|   TEXAS INSTRUMENTS INCORPORATED
|   Standard Linear and Logic
|   IBIS Model of SN74LVTH16652
|   3.3-V ABT 16-BIT BUS TRANSCEIVERS AND REGISTERS
|   WITH 3-STATE OUTPUTS
|   TSSOP 56-pin package (DGG)
|   SSOP 56-pin package (DL)
[IBIS Ver]   3.2
[Comment char] |_char
[File Name]   sn74lvth16652.ibs
[File Rev]   1.1 | x_rev
[Date]   10/03/03
[Source]   File originated at Texas Instruments, Inc
[Notes]   The following is a sample IBIS file for the SN74LVTH16652.
|   - All test data contained in this file are derived from
|   actual measurement.
|   - The measurement used DGG package.
|   - We have data across voltage and temperature, but not across
|   process.
|   - Since this is a BiCMOS process, we have irregular trend for the
|   curves at high and low temperatures. This data was taken with
|   high temperature for strong case and low for weak case.
|   - Due to presence of BUS-HOLD at input, GND-CLAMP curves
|   have non-monotonic warnings.
|   - End point warning due to AC and DC mismatch.
|   - Due to the fact that the Device is 5-V Input/Output
|   tolarent, the I/O model has some Non-Monotonic Warnings.
|   - File created by Nobuhisa Ohtsubo, TIJ SLL Product Engineering.
|*   Property of Texas Instruments Incorporated.  Unauthorized   *
|*   reproduction and/or distribution is strictly prohibited.   *
|*   This product is protected under copyright law.   *
|*   Created 1998, (C) Copyright 1998, Texas Instruments Inc.,   *
|*   All Rights Reserved   *
|*   UNLESS THERE IS A SIGNED, WRITTEN AGREEMENT TO THE   *
|*   CONTRARY, TEXAS INSTRUMENTS ("TI") IS PROVIDING THE SPICE   *
|*   MODELS "AS IS" AND WITHOUT ANY WARRANTY, EXPRESSED OR   *
|*   IMPLIED.  TI assumes no liability for:   *
|*   1) the accuracy of the IBIS models provided to your   *
|*   company;   *
|*   2) the proper functioning of these IBIS models in your   *
|*   design or for any resulting applications; or   *
|*   3) infringement of patents, copyrights or intellectual   *
|*   property rights resulting from your use of these   *
|*   IBIS models.   *
|*   TI provides IBIS Models as a service to our customers.   *
|*   You and your company shall not distribute, sell or give   *
|*   these models to anyone else without prior written   *
|*   permission from TI.   *
|*   TI reserves the right to make changes to our products or   *
|*   to discontinue any semiconductor product or service   *
|*   without notice, and advises our customers to obtain the   *
|*   latest version of relevant information to verify, before   *
|*   placing orders, that the information being relied on is   *
|*   current.   *
|*   Please be aware that your receipt and use of the IBIS   *
|*   information provided shall serve as acceptance of these   *
|*   terms and conditions.  If you do not accept these terms,   *
|*   you should return or destroy the IBIS models and any   *
|*   other accompanying information immediately.   *
|   TSSOP PACKAGE (DGG)
[Component]   LVTH16652_DGG
[manufacturer]   Texas Instruments, Inc.
[Package]
|   typ   min   max
R_pkg   0.045   0.035   0.062
L_pkg   3.324nH   2.403nH   5.094nH
C_pkg   0.564pF   0.341pF   0.914nH
[Pin] signal_name   model_name   R_pin   L_pin   C_pin
1   1OEAB   LVTH16652_CTRL   0.062   5.094nH   0.856pF
2   1CLKAB   LVTH16652_CTRL   0.061   4.621nH   0.902pF
3   1SAB   LVTH16652_CTRL   0.060   4.316nH   0.802pF
4   GND   GND   0.059   3.968nH   0.698pF
5   1A1   LVTH16652_IO   0.057   3.716nH   0.649pF
6   1A2   LVTH16652_IO   0.042   3.517nH   0.652pF
7   VCC   POWER   0.041   3.160nH   0.570pF
8   1A3   LVTH16652_IO   0.039   2.981nH   0.482pF
9   1A4   LVTH16652_IO   0.039   2.809nH   0.447pF
10   1A5   LVTH16652_IO   0.038   2.715nH   0.409pF
11   GND   GND   0.041   2.675nH   0.391pF
12   1A6   LVTH16652_IO   0.039   2.536nH   0.366pF
13   1A7   LVTH16652_IO   0.039   2.457nH   0.348pF
14   1A8   LVTH16652_IO   0.038   2.411nH   0.353pF
15   2A1   LVTH16652_IO   0.039   2.456nH   0.355pF
16   2A2   LVTH16652_IO   0.039   2.471nH   0.349pF
17   2A3   LVTH16652_IO   0.040   2.580nH   0.370pF
18   GND   GND   0.038   2.651nH   0.389pF
19   2A4   LVTH16652_IO   0.038   2.739nH   0.411pF
20   2A5   LVTH16652_IO   0.039   2.838nH   0.449pF
21   2A6   LVTH16652_IO   0.038   2.988nH   0.484pF
22   VCC   POWER   0.038   3.105nH   0.564pF
23   2A7   LVTH16652_IO   0.040   3.427nH   0.638pF
24   2A8   LVTH16652_IO   0.056   3.654nH   0.641pF
25   GND   GND   0.057   3.932nH   0.700pF
26   2SAB   LVTH16652_CTRL   0.058   4.257nH   0.806pF
27   2CLKAB   LVTH16652_CTRL   0.057   4.580nH   0.914pF
28   2OEAB   LVTH16652_CTRL   0.059   5.038nH   0.861pF
29   2OEBA_BAR   LVTH16652_CTRL   0.060   5.058nH   0.858pF
30   2CLKBA   LVTH16652_CTRL   0.056   4.543nH   0.904pF
31   2SBA   LVTH16652_CTRL   0.057   4.240nH   0.803pF
32   GND   GND   0.057   3.929nH   0.700pF
33   2B8   LVTH16652_IO   0.056   3.616nH   0.637pF
34   2B7   LVTH16652_IO   0.037   3.368nH   0.640pF
35   VCC   POWER   0.036   3.024nH   0.563pF
36   2B6   LVTH16652_IO   0.035   2.876nH   0.474pF
37   2B5   LVTH16652_IO   0.035   2.745nH   0.444pF
38   2B4   LVTH16652_IO   0.037   2.683nH   0.405pF
39   GND   GND   0.038   2.603nH   0.382pF
40   2B3   LVTH16652_IO   0.038   2.510nH   0.362pF
41   2B2   LVTH16652_IO   0.036   2.412nH   0.341pF
42   2B1   LVTH16652_IO   0.038   2.416nH   0.349pF
43   1B8   LVTH16652_IO   0.037   2.403nH   0.349pF
44   1B7   LVTH16652_IO   0.037   2.429nH   0.341pF
45   1B6   LVTH16652_IO   0.036   2.482nH   0.358pF
46   GND   GND   0.037   2.615nH   0.381pF
47   1B5   LVTH16652_IO   0.035   2.669nH   0.402pF
48   1B4   LVTH16652_IO   0.036   2.763nH   0.442pF
49   1B3   LVTH16652_IO   0.036   2.942nH   0.478pF
50   VCC   POWER   0.035   3.053nH   0.564pF
51   1B2   LVTH16652_IO   0.036   3.409nH   0.641pF
52   1B1   LVTH16652_IO   0.058   3.698nH   0.641pF
53   GND   GND   0.059   3.975nH   0.697pF
54   1SBA   LVTH16652_CTRL   0.061   4.327nH   0.802pF
55   1CLKBA   LVTH16652_CTRL   0.061   4.624nH   0.905pF
56   1OEBA_BAR   LVTH16652_CTRL   0.060   5.063nH   0.858pF
|   SSOP PACKAGE (DL)
[Component]   LVTH16652_DL
[manufacturer]   Texas Instruments, Inc.
[Package]
|   typ   min   max
R_pkg   0.055   0.048   0.067
L_pkg   6.539nH   4.802nH   9.746nH
C_pkg   0.85pF   0.5pF   1.351pF
[Pin] signal_name   model_name   R_pin   L_pin   C_pin
1   1OEAB   LVTH16652_CTRL   0.064   9.646nH   1.202pF
2   1CLKAB   LVTH16652_CTRL   0.059   8.723nH   1.348pF
3   1SAB   LVTH16652_CTRL   0.059   8.139nH   1.223pF
4   GND   GND   0.056   7.554nH   1.088pF
5   1A1   LVTH16652_IO   0.054   6.991nH   0.966pF
6   1A2   LVTH16652_IO   0.053   6.659nH   0.973pF
7   VCC   POWER   0.055   6.321nH   0.905pF
8   1A3   LVTH16652_IO   0.055   5.942nH   0.713pF
9   1A4   LVTH16652_IO   0.057   5.767nH   0.678pF
10   1A5   LVTH16652_IO   0.054   5.459nH   0.631pF
11   GND   GND   0.051   5.224nH   0.638pF
12   1A6   LVTH16652_IO   0.048   5.088nH   0.601pF
13   1A7   LVTH16652_IO   0.050   5.021nH   0.518pF
14   1A8   LVTH16652_IO   0.051   4.802nH   0.500pF
15   2A1   LVTH16652_IO   0.051   4.803nH   0.500pF
16   2A2   LVTH16652_IO   0.050   5.021nH   0.518pF
17   2A3   LVTH16652_IO   0.048   5.088nH   0.601pF
18   GND   GND   0.051   5.224nH   0.638pF
19   2A4   LVTH16652_IO   0.054   5.459nH   0.631pF
20   2A5   LVTH16652_IO   0.057   5.768nH   0.677pF
21   2A6   LVTH16652_IO   0.055   5.942nH   0.715pF
22   VCC   POWER   0.055   6.321nH   0.907pF
23   2A7   LVTH16652_IO   0.053   6.659nH   0.972pF
24   2A8   LVTH16652_IO   0.054   6.991nH   0.966pF
25   GND   GND   0.056   7.554nH   1.087pF
26   2SAB   LVTH16652_CTRL   0.059   8.139nH   1.223pF
27   2CLKAB   LVTH16652_CTRL   0.059   8.727nH   1.351pF
28   2OEAB   LVTH16652_CTRL   0.067   9.746nH   1.210pF
29   2OEBA_BAR   LVTH16652_CTRL   0.063   9.630nH   1.203pF
30   2CLKBA   LVTH16652_CTRL   0.060   8.751nH   1.349pF
31   2SBA   LVTH16652_CTRL   0.060   8.184nH   1.224pF
32   GND   GND   0.056   7.543nH   1.087pF
33   2B8   LVTH16652_IO   0.054   7.005nH   0.969pF
34   2B7   LVTH16652_IO   0.056   6.714nH   0.975pF
35   VCC   POWER   0.058   6.384nH   0.909pF
36   2B6   LVTH16652_IO   0.057   5.976nH   0.717pF
37   2B5   LVTH16652_IO   0.057   5.743nH   0.677pF
38   2B4   LVTH16652_IO   0.055   5.469nH   0.631pF
39   GND   GND   0.055   5.328nH   0.644pF
40   2B3   LVTH16652_IO   0.052   5.189nH   0.606pF
41   2B2   LVTH16652_IO   0.052   5.053nH   0.519pF
42   2B1   LVTH16652_IO   0.052   4.825nH   0.502pF
43   1B8   LVTH16652_IO   0.054   4.896nH   0.506pF
44   1B7   LVTH16652_IO   0.052   5.093nH   0.521pF
45   1B6   LVTH16652_IO   0.051   5.179nH   0.608pF
46   GND   GND   0.054   5.314nH   0.645pF
47   1B5   LVTH16652_IO   0.055   5.511nH   0.632pF
48   1B4   LVTH16652_IO   0.057   5.770nH   0.677pF
49   1B3   LVTH16652_IO   0.055   5.956nH   0.716pF
50   VCC   POWER   0.055   6.320nH   0.905pF
51   1B2   LVTH16652_IO   0.052   6.621nH   0.968pF
52   1B1   LVTH16652_IO   0.053   6.974nH   0.966pF
53   GND   GND   0.057   7.571nH   1.089pF
54   1SBA   LVTH16652_CTRL   0.057   8.097nH   1.219pF
55   1CLKBA   LVTH16652_CTRL   0.059   8.723nH   1.349pF
56   1OEBA_BAR   LVTH16652_CTRL   0.061   9.560nH   1.199pF
[Model Selector]   LVTH16652_IO
LVTH16652_IO_28   2.8-V Vcc Input/Output Model
LVTH16652_IO_33   3.3-V Vcc Input/Output Model
[Model Selector]   LVTH16652_CTRL
LVTH16652_CTRL_28   2.8-V Vcc Input Model
LVTH16652_CTRL_33   3.3-V Vcc Input Model
| Models and submodels in the file (4): LVTH16652_IO_28 (I/O), LVTH16652_CTRL_28 (Input), LVTH16652_IO_33 (I/O), LVTH16652_CTRL_33 (Input)
